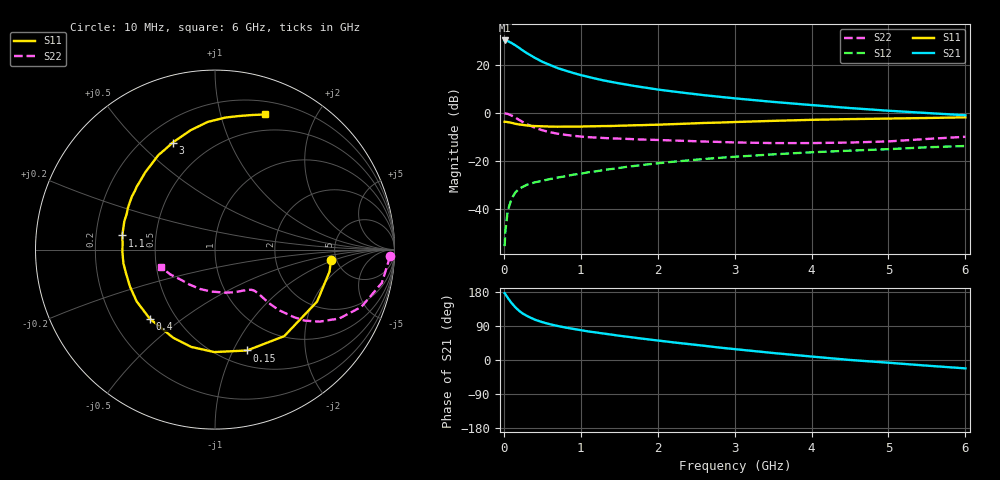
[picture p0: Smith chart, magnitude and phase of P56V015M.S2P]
! SIEMENS Small Signal Semiconductors
! BFP183
! Si NPN RF Bipolar Junction Transistor in SOT143
! VCE = 6 V  IC = 15 mA
! Common Emitter S-Parameters:  March  1996
# GHz  S  MA  R  50
!  f  S11  S21  S12  S22
! GHz  MAG  ANG  MAG  ANG  MAG  ANG  MAG  ANG
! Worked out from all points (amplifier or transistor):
!   36 points, 10 MHz to 6 GHz, reference 50 ohm
!   highest |S21| = 30.0 dB at 10 MHz (marker M1)
!   |S21| within 3 dB of that: start of sweep to 195.6 MHz
!   unconditionally stable (mu >= 1): 998.9 MHz to 5.669 GHz
!   at 250 MHz: K = 0.39, MSG = 28.2 dB, |S12| = -30.7 dB
!   at 1.4 GHz: K = 1.10, MAG = 16.1 dB, |S12| = -23.4 dB
!   at 6 GHz: K = 0.96, MSG = 6.4 dB, |S12| = -13.8 dB
!   S11 on the Smith chart (normalised r, x): 10 MHz: 4.51, -0.92; 150 MHz: 0.66, -1.13; 400 MHz: 0.36, -0.38; 1.1 GHz: 0.32, +0.07; 3 GHz: 0.31, +0.63; 6 GHz: 0.33, +1.39
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0.01  0.6492 -5.2  31.65 176.5  0.0017 83.4  0.9761 -2.2
0.02  0.6496 -10.9  31.52 173.7  0.0035 89.9  0.9667 -4.5
0.05  0.6383 -27.0  30.77 164.3  0.0091 81.1  0.948 -11.3
0.1  0.6175 -51.3  28.08 150.6  0.0164 67.9  0.8756 -21.4
0.15  0.5897 -72.4  25.04 138.9  0.0222 61.1  0.7917 -29.0
0.2  0.5709 -90.4  22.17 129.5  0.0266 55.3  0.7086 -34.5
0.25  0.5582 -103.7  19.42 122.1  0.0291 51.7  0.6371 -38.4
0.3  0.5436 -115.4  17.28 116.4  0.0321 49.3  0.5776 -40.6
0.4  0.5294 -133.4  13.9 106.7  0.0358 46.5  0.4912 -43.4
0.5  0.5232 -146.6  11.45 99.9  0.0388 45.7  0.4327 -44.6
0.6  0.5165 -156.5  9.806 94.4  0.042 45.8  0.3939 -45.0
0.7  0.5131 -165.0  8.447 89.8  0.0452 46.5  0.3673 -45.2
0.9  0.5161 -178.4  6.719 82.2  0.0517 47.4  0.333 -45.7
1.1  0.5225 171.3  5.538 75.3  0.0581 48.1  0.3114 -46.7
1.5  0.5377 154.6  4.072 64.0  0.0716 48.5  0.2902 -50.6
1.8  0.5529 143.9  3.393 56.3  0.0823 47.7  0.2778 -55.1
2.2  0.5801 132.1  2.763 46.6  0.0961 45.4  0.2654 -62.2
3  0.6412 111.6  1.992 28.7  0.1219 39.8  0.2417 -80.7
3.5  0.6785 101.6  1.68 18.5  0.1368 35.9  0.2346 -94.6
4.5  0.7377 85.6  1.251 0.1  0.1634 27.6  0.2409 -125.8
5.5  0.7778 74.6  0.987 -14.9  0.1919 20.3  0.2857 -151.2
6  0.8031 69.6  0.887 -22.1  0.2041 15.9  0.3169 -162.5
